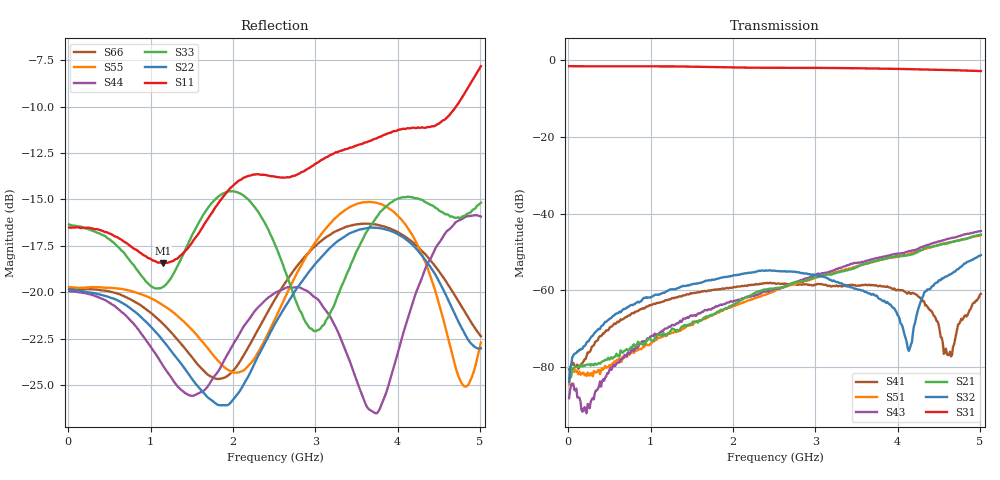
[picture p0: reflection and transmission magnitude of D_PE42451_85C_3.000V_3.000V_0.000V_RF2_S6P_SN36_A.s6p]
! Device ID: PE42451
! Serial: 36
! Insertion: A
! Temp: 85C
! VDD: 3.000
! Control_Hi: 100.000
! Control_Lo: 0.000
! Logic State: RF2
! Port 1: RFC
! Port 2: RF1
! Port 3: RF2
! Port 4: RF3
! Port 5: RF4
! Port 6: RF5
! V1 = 0.00
! V2 = 3.00
! V3 = 0.00
! V4 = 0.00
! IDD: 1.419120e-05
#  Hz  S  RI  R  50
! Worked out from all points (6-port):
!   401 points, 10 MHz to 5.01 GHz, reference 50 ohm
!   strongest paths, dB at 10 MHz, 1.26 GHz, 2.51 GHz, 3.76 GHz, 5.01 GHz:
!     S31: -1.6, -1.6, -2.0, -2.2, -2.8
!     S32: -83.9, -59.8, -54.9, -62.0, -50.9
!     S21: -82.9, -70.0, -59.5, -52.3, -45.5
!     S43: -88.1, -69.0, -59.6, -51.6, -44.5
!     S51: -84.5, -71.1, -60.2, -52.2, -45.6
!     S41: -80.6, -62.0, -58.2, -59.0, -61.0
!   lowest |S11| = -18.4 dB at 1.147 GHz (marker M1), VSWR 1.27, Z = 58.1 - j10.1 ohm
!   |S11| at or under -10 dB: start of sweep to 4.708 GHz
